(* Logix 5000 AddOnInstructionDefinition export Banner_K30Pro_PD_v4; software revision 33.00 *)

TYPE Banner_K30Pro_4State_v4 :   // Process Data for Four Staet Mode. This mode is only available in Touch models.
STRUCT
   Touch_Status : SINT;   // 0 = Inactive, 1 = Active. Only active for Touch models.
   In_State : SINT;   // Curent State. 0 = State 1, 1 = State 2, 2 = State 3, 3 = State 4
   Job_Control : SINT;   // 0 = Off, 1 = On
END_STRUCT
END_TYPE

TYPE Banner_K30Pro_Adv_v4 :   // Advanced Process Data information for a Banner K30 Pro.
STRUCT
   Touch_Status : SINT;   // 0 = Inactive, 1 = Active. Only active for Touch models.
   Type : SINT;   // 0 = Off, 1 = Steady, 2 = Flash, 3 = Two Color Flash, 4 = 50/50, 5 = 50/50 Rotate, 6 = Chase, 7 = Intensity Sweep, 8 = Sequence.
   Direction : SINT;   // 0 = CCW, 1 = CW.
   Pattern : SINT;   // 0 = Flash, 1 = Strobe, 2 = Three Pulse, 3 = SOS, 4 = Random.
   Speed : SINT;   // 0 = Slow, 1 = Medium, 2 = Fast, 3 = Custom.
   Reserved : SINT;
   Dynamic_Sequence : INT;   // 0 to 255. Value describing the LED position on the device.
   Sequence_Start_Location : SINT;   // 0 = LED 1, 1 = LED 2, 2 = LED 3, 3 = LED 4.
   Color_1 : SINT;   // 0 = Green, 1 = Red, 2 = Orange, 3 = Amber, 4 = Yellow, 5 = Lime Green, 6 = Spring Green, 7 = Cyan, 8 = Sky Blue, 9 = Blue, 10 = Violet, 11 = Magenta, 12 = Rose, 13 = White, 14 = Custom 1, 15 = Custom 2.
   Color_1_Intensity : SINT;   // 0 = High, 1 = Medium, 2 = Low, 3 = Off, 4 = Custom.
   Color_2 : SINT;   // 0 = Green, 1 = Red, 2 = Orange, 3 = Amber, 4 = Yellow, 5 = Lime Green, 6 = Spring Green, 7 = Cyan, 8 = Sky Blue, 9 = Blue, 10 = Violet, 11 = Magenta, 12 = Rose, 13 = White, 14 = Custom 1, 15 = Custom 2.
   Color_2_Intensity : SINT;   // 0 = High, 1 = Medium, 2 = Low, 3 = Off, 4 = Custom.
END_STRUCT
END_TYPE

TYPE Banner_K30Pro_LED_v4 :   // LED Control Process Data for a K30 Pro Touch.
STRUCT
   Touch_Status : SINT;   // 0 = Inactive, 1 = Active. Only active for Touch models.
   LED_1_Color : SINT;   // 0 = Green, 1 = Red, 2 = Orange, 3 = Amber, 4 = Yellow, 5 = Lime Green, 6 = Spring Green, 7 = Cyan, 8 = Sky Blue, 9 = Blue, 10 = Violet, 11 = Magenta, 12 = Rose, 13 = White, 14 = Custom 1, 15 = Custom 2.
   LED_1_Intensity : SINT;   // 0 to 10 (0 to 100%).
   LED_2_Color : SINT;   // 0 = Green, 1 = Red, 2 = Orange, 3 = Amber, 4 = Yellow, 5 = Lime Green, 6 = Spring Green, 7 = Cyan, 8 = Sky Blue, 9 = Blue, 10 = Violet, 11 = Magenta, 12 = Rose, 13 = White, 14 = Custom 1, 15 = Custom 2.
   LED_2_Intensity : SINT;   // 0 to 10 (0 to 100%).
   LED_3_Color : SINT;   // 0 = Green, 1 = Red, 2 = Orange, 3 = Amber, 4 = Yellow, 5 = Lime Green, 6 = Spring Green, 7 = Cyan, 8 = Sky Blue, 9 = Blue, 10 = Violet, 11 = Magenta, 12 = Rose, 13 = White, 14 = Custom 1, 15 = Custom 2.
   LED_3_Intensity : SINT;   // 0 to 10 (0 to 100%).
   LED_4_Color : SINT;   // 0 = Green, 1 = Red, 2 = Orange, 3 = Amber, 4 = Yellow, 5 = Lime Green, 6 = Spring Green, 7 = Cyan, 8 = Sky Blue, 9 = Blue, 10 = Violet, 11 = Magenta, 12 = Rose, 13 = White, 14 = Custom 1, 15 = Custom 2.
   LED_4_Intensity : SINT;   // 0 to 10 (0 to 100%).
END_STRUCT
END_TYPE

TYPE Banner_K30Pro_MC_v4 :   // Process Data for Multicolor
STRUCT
   Touch_Status : SINT;   // 0 = Inactive, 1 = Active. Only active for Touch models.
   In_State : SINT;   // Curent State. 0 = State 1, 1 = State 2, 2 = State 3, 3 = State 4
   Out_State : SINT;   // Set Output State. 0 = State 1, 1 = State 2, 2 = State 3, 3 = State 4
END_STRUCT
END_TYPE

TYPE Banner_K30Pro_PDIO_v4 :   // UDT that records the converted prcoess data.
STRUCT
   PD_MultiColor_State : Banner_K30Pro_MC_v4;   // Only active when Operation Mode set to 0.
   PD_Four_State : Banner_K30Pro_4State_v4;   // Only active when Operation Mode set to 1. Only available in Touch models.
   PD_Advanced : Banner_K30Pro_Adv_v4;   // Only active when Operation Mode set to 2.
   PD_LED : Banner_K30Pro_LED_v4;   // Only active when Operation Mode set to 3.
   PDO_DT : SINT[10];
   PDI_DT : SINT[2];
END_STRUCT
END_TYPE

ADD_ON_INSTRUCTION Banner_K30Pro_PD_v4   (* revision 4.0, vendor Banner Engineering *)
// Takes the raw SINT information and converts that data into actual information.
VAR_IN_OUT
   Process_Data : Banner_K30Pro_PDIO_v4; {required}
END_VAR
VAR_INPUT
   Operation_Mode : SINT; {required}   // Linked from Parameters AOI or entered manually.
   Byte_Swap : BOOL; {required}
END_VAR
VAR
   PDO_Temp : SINT[10]; {access None}
   PDI_Temp : SINT[2]; {access None}
END_VAR

ROUTINE Logic   (* ladder *)
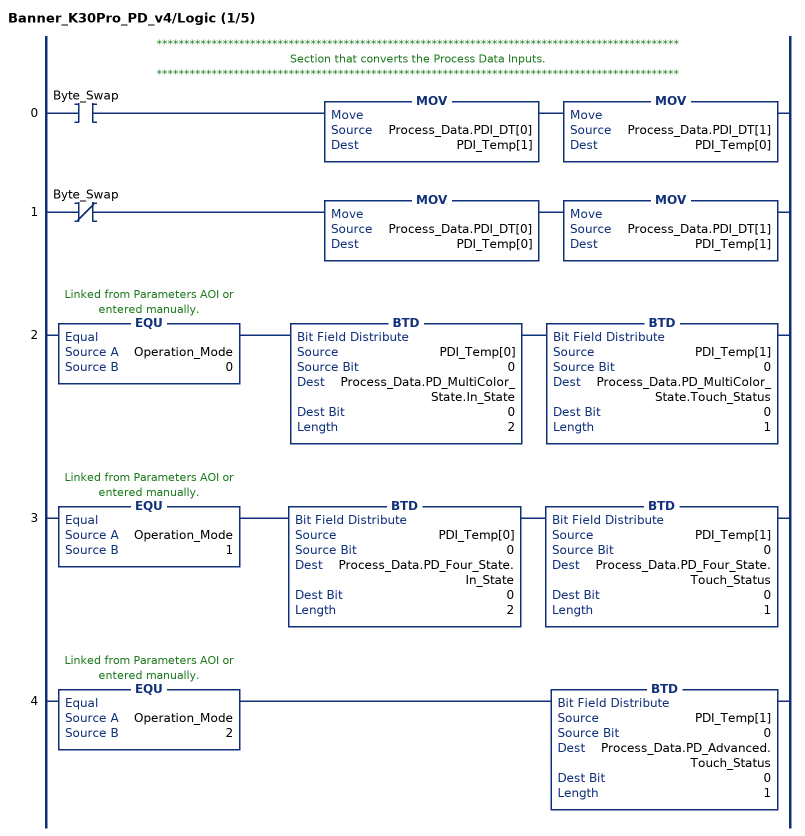
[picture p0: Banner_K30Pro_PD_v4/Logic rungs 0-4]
   // ***********************************************************************************************
   // Section that converts the Process Data Inputs.
   // ***********************************************************************************************
   0: XIC(Byte_Swap)MOV(Process_Data.PDI_DT[0],PDI_Temp[1])MOV(Process_Data.PDI_DT[1],PDI_Temp[0]);
   1: XIO(Byte_Swap)MOV(Process_Data.PDI_DT[0],PDI_Temp[0])MOV(Process_Data.PDI_DT[1],PDI_Temp[1]);
   2: EQU(Operation_Mode,0)BTD(PDI_Temp[0],0,Process_Data.PD_MultiColor_State.In_State,0,2)BTD(PDI_Temp[1],0,Process_Data.PD_MultiColor_State.Touch_Status,0,1);
   3: EQU(Operation_Mode,1)BTD(PDI_Temp[0],0,Process_Data.PD_Four_State.In_State,0,2)BTD(PDI_Temp[1],0,Process_Data.PD_Four_State.Touch_Status,0,1);
   4: EQU(Operation_Mode,2)BTD(PDI_Temp[1],0,Process_Data.PD_Advanced.Touch_Status,0,1);
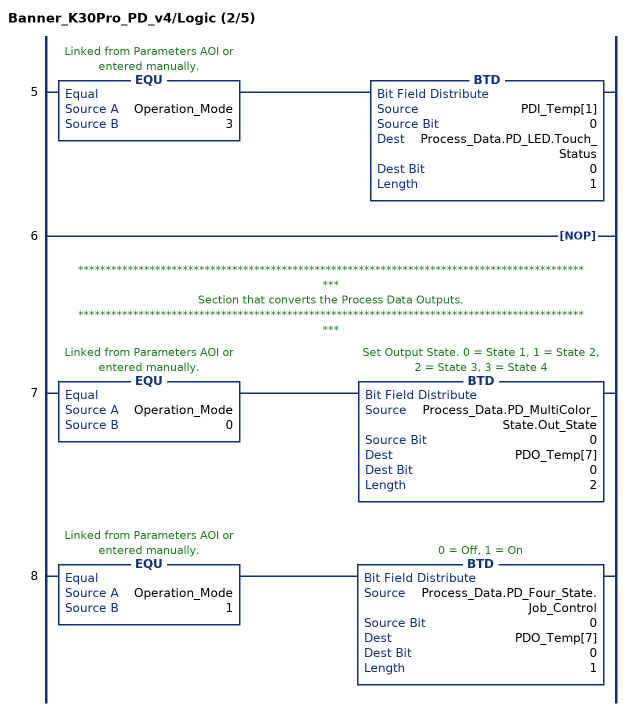
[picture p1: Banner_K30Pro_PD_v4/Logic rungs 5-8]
   5: EQU(Operation_Mode,3)BTD(PDI_Temp[1],0,Process_Data.PD_LED.Touch_Status,0,1);
   6: NOP();
   // ***********************************************************************************************
   // Section that converts the Process Data Outputs.
   // ***********************************************************************************************
   7: EQU(Operation_Mode,0)BTD(Process_Data.PD_MultiColor_State.Out_State,0,PDO_Temp[7],0,2);
   8: EQU(Operation_Mode,1)BTD(Process_Data.PD_Four_State.Job_Control,0,PDO_Temp[7],0,1);
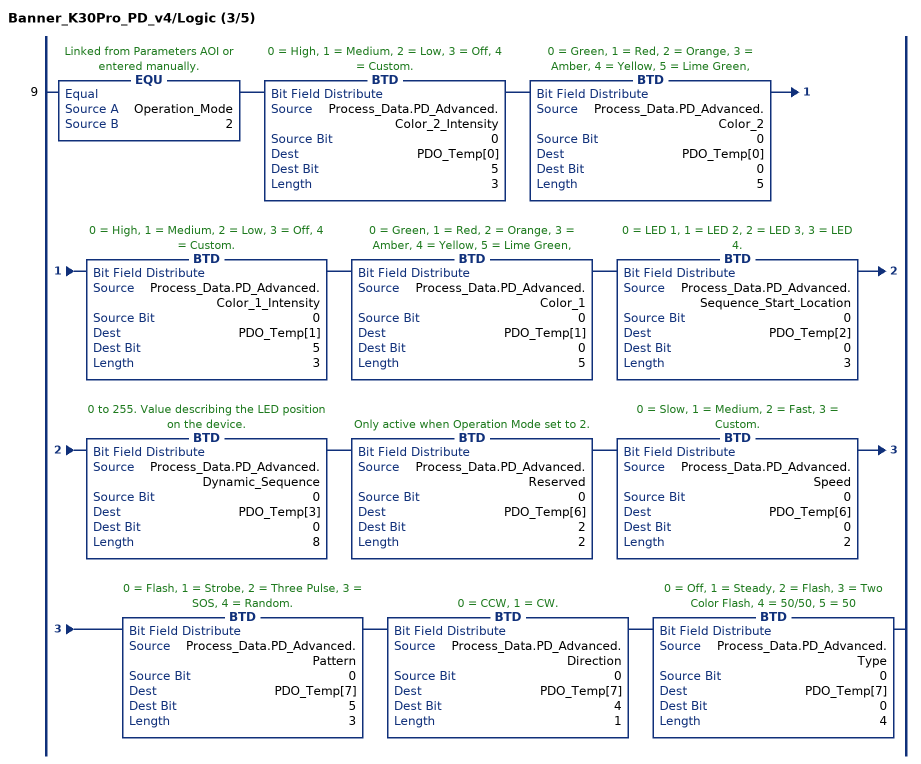
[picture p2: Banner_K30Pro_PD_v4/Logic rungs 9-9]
   9: EQU(Operation_Mode,2)BTD(Process_Data.PD_Advanced.Color_2_Intensity,0,PDO_Temp[0],5,3)BTD(Process_Data.PD_Advanced.Color_2,0,PDO_Temp[0],0,5)BTD(Process_Data.PD_Advanced.Color_1_Intensity,0,PDO_Temp[1],5,3)BTD(Process_Data.PD_Advanced.Color_1,0,PDO_Temp[1],0,5)BTD(Process_Data.PD_Advanced.Sequence_Start_Location,0,PDO_Temp[2],0,3)BTD(Process_Data.PD_Advanced.Dynamic_Sequence,0,PDO_Temp[3],0,8)BTD(Process_Data.PD_Advanced.Reserved,0,PDO_Temp[6],2,2)BTD(Process_Data.PD_Advanced.Speed,0,PDO_Temp[6],0,2)BTD(Process_Data.PD_Advanced.Pattern,0,PDO_Temp[7],5,3)BTD(Process_Data.PD_Advanced.Direction,0,PDO_Temp[7],4,1)BTD(Process_Data.PD_Advanced.Type,0,PDO_Temp[7],0,4);
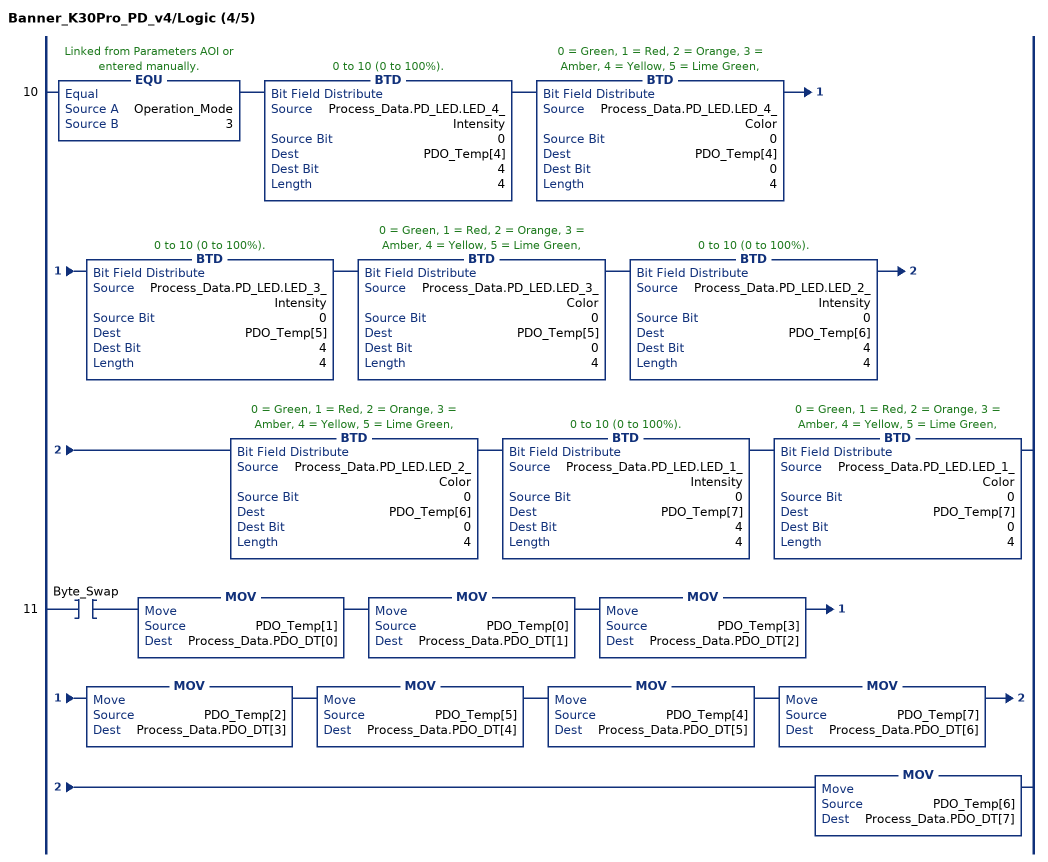
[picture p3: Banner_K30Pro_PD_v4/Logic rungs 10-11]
   10: EQU(Operation_Mode,3)BTD(Process_Data.PD_LED.LED_4_Intensity,0,PDO_Temp[4],4,4)BTD(Process_Data.PD_LED.LED_4_Color,0,PDO_Temp[4],0,4)BTD(Process_Data.PD_LED.LED_3_Intensity,0,PDO_Temp[5],4,4)BTD(Process_Data.PD_LED.LED_3_Color,0,PDO_Temp[5],0,4)BTD(Process_Data.PD_LED.LED_2_Intensity,0,PDO_Temp[6],4,4)BTD(Process_Data.PD_LED.LED_2_Color,0,PDO_Temp[6],0,4)BTD(Process_Data.PD_LED.LED_1_Intensity,0,PDO_Temp[7],4,4)BTD(Process_Data.PD_LED.LED_1_Color,0,PDO_Temp[7],0,4);
   11: XIC(Byte_Swap)MOV(PDO_Temp[1],Process_Data.PDO_DT[0])MOV(PDO_Temp[0],Process_Data.PDO_DT[1])MOV(PDO_Temp[3],Process_Data.PDO_DT[2])MOV(PDO_Temp[2],Process_Data.PDO_DT[3])MOV(PDO_Temp[5],Process_Data.PDO_DT[4])MOV(PDO_Temp[4],Process_Data.PDO_DT[5])MOV(PDO_Temp[7],Process_Data.PDO_DT[6])MOV(PDO_Temp[6],Process_Data.PDO_DT[7]);
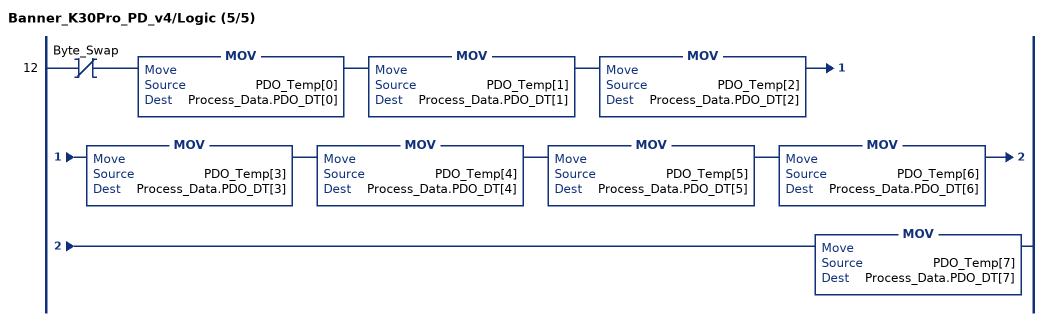
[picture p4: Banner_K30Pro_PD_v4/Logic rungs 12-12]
   12: XIO(Byte_Swap)MOV(PDO_Temp[0],Process_Data.PDO_DT[0])MOV(PDO_Temp[1],Process_Data.PDO_DT[1])MOV(PDO_Temp[2],Process_Data.PDO_DT[2])MOV(PDO_Temp[3],Process_Data.PDO_DT[3])MOV(PDO_Temp[4],Process_Data.PDO_DT[4])MOV(PDO_Temp[5],Process_Data.PDO_DT[5])MOV(PDO_Temp[6],Process_Data.PDO_DT[6])MOV(PDO_Temp[7],Process_Data.PDO_DT[7]);
END_ROUTINE
END_ADD_ON_INSTRUCTION
